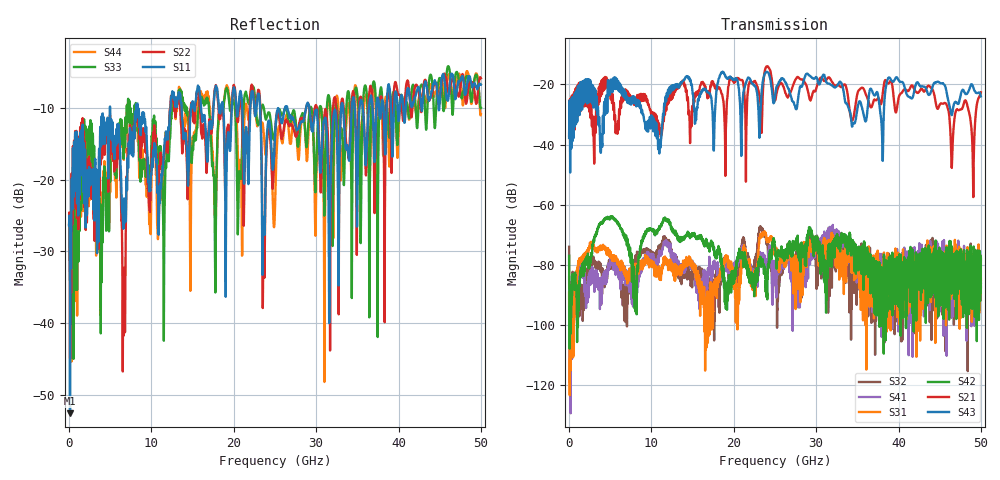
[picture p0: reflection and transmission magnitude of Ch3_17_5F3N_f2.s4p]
!Agilent Technologies,N5247A,US51170199,A.09.90.13
!Agilent N5247A: A.09.90.13
!Date: Wednesday, December 09, 2015 09:35:03
!Correction: S11(Full 4 Port(1,2,3,4))
!S12(Full 4 Port(1,2,3,4))
!S13(Full 4 Port(1,2,3,4))
!S14(Full 4 Port(1,2,3,4))
!S21(Full 4 Port(1,2,3,4))
!S22(Full 4 Port(1,2,3,4))
!S23(Full 4 Port(1,2,3,4))
!S24(Full 4 Port(1,2,3,4))
!S31(Full 4 Port(1,2,3,4))
!S32(Full 4 Port(1,2,3,4))
!S33(Full 4 Port(1,2,3,4))
!S34(Full 4 Port(1,2,3,4))
!S41(Full 4 Port(1,2,3,4))
!S42(Full 4 Port(1,2,3,4))
!S43(Full 4 Port(1,2,3,4))
!S44(Full 4 Port(1,2,3,4))
!S4P File: Measurements: <S11,S12,S13,S14>,
!<S21,S22,S23,S24>,
!<S31,S32,S33,S34>,
!<S41,S42,S43,S44>:
# Hz S  dB  R 50
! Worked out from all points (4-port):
!   3201 points, 10 MHz to 50 GHz, reference 50 ohm
!   strongest paths, dB at 10 MHz, 12.51 GHz, 25 GHz, 37.5 GHz, 50 GHz:
!     S43: -37.8, -20.4, -23.9, -23.4, -23.9
!     S21: -37.0, -22.5, -25.2, -24.6, -22.6
!     S42: -77.0, -68.7, -74.0, -86.0, -77.9
!     S31: -89.2, -82.1, -75.1, -82.1, -85.0
!     S41: -84.1, -76.8, -82.4, -81.3, -85.9
!     S32: -73.9, -78.6, -81.3, -93.8, -87.4
!   lowest |S11| = -52.6 dB at 119.4 MHz (marker M1), VSWR 1.00, Z = 50 + j0.231 ohm
!   |S11| at or under -10 dB: start of sweep to 4.96 GHz; 8.347 GHz to 12.32 GHz (3.973 GHz wide, 38.4 % of centre); 29.17 GHz to 33.03 GHz (3.857 GHz wide, 12.4 % of centre)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
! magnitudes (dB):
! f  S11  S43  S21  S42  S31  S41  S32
! 10 MHz  -26.4  -37.8  -37.0  -77.0  -89.2  -84.1  -73.9
! 119.4 MHz  -52.6  -34.6  -36.2  -93.8  -95.9  -97.9  -92.6
! 5.118 GHz  -11.6  -22.2  -22.5  -64.1  -77.7  -79.4  -78.7
! 6.649 GHz  -24.3  -24.2  -23.3  -69.7  -82.6  -82.3  -88.2
! 24.08 GHz  -12.9  -15.9  -13.9  -84.2  -72.3  -81.3  -73.2
! 49.05 GHz  -6.8  -20.7  -51.0  -78.7  -76.5  -88.5  -87.2
! 50 GHz  -6.7  -23.9  -22.6  -77.9  -85.0  -85.9  -87.4
